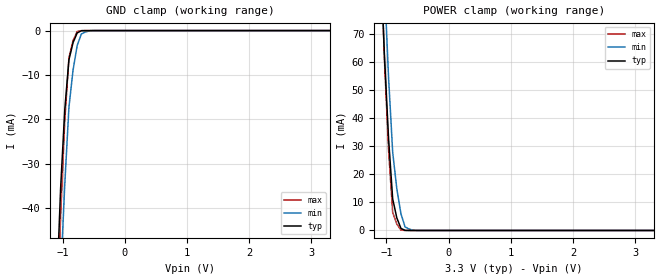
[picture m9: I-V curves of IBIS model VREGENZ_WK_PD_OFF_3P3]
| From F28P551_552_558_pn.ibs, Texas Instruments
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|   Model Cell VREGENZ_WK_PD_OFF_3P3
|VREGENZ_WK_PD_OFF_3P3
[Model]   VREGENZ_WK_PD_OFF_3P3
Model_type   Input
Polarity   Non-Inverting
Vinl =  0.8
Vinh =  2
C_comp   1.1812p   1.10922p   1.21731p
[Model Spec]
Vinl   0.8   0.8   0.8
Vinh   2   2   2
[Temperature Range]   25   155   -40
[Voltage Range]   3.3   2.97   3.63
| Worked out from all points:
|   GND clamp passes 1 mA (typ) near -0.78 V on its own axis
|   POWER clamp passes 1 mA (typ) near -0.77 V on its own axis
| Nom Voltages:
|   BIASFET=3.3, VDD=1.2, VDDS=3.3, VSS=0
| Min Voltages:
|   BIASFET=2.97, VDD=1.08, VDDS=2.97, VSS=0
| Max Voltages:
|   BIASFET=3.63, VDD=1.32, VDDS=3.63, VSS=0
[POWER_clamp]
|   voltage   I(typ)   I(min)   I(max)
-3.3V     1.823A     2.351A     1.96A
-1.1V     100.7mA    129.7mA    103.9mA
-1.033V   62.81mA    88.77mA    61.28mA
-966.7mV  33mA       54.86mA    28.79mA
-900mV    11.27mA    27.96mA    6.481mA
-833.3mV  4.489mA    14.84mA    2.278mA
-766.7mV  744.5uA    5.933mA    118.9uA
-700mV    35.91uA    1.232mA    3.424uA
-566.7mV  940.6nA    77.14uA    314.2nA
3.3V      -122.2pA   -177.2nA   -105pA
[GND_clamp]
|   voltage   I(typ)   I(min)   I(max)
-3.3V     -1.38A     -1.323A    -2.074A
-1.1V     -59.59mA   -79.11mA   -70.71mA
-1.033V   -35.48mA   -55.25mA   -41.82mA
-966.7mV  -17.81mA   -34.65mA   -20.29mA
-900mV    -6.579mA   -17.32mA   -6.122mA
-833.3mV  -2.708mA   -8.854mA   -2.234mA
-766.7mV  -527.3uA   -3.335mA   -196uA
-700mV    -37.18uA   -766.2uA   -8.209uA
-566.7mV  -1.613uA   -62.25uA   -984.8nA
3.3V      175pA      136.4nA    162.8pA
